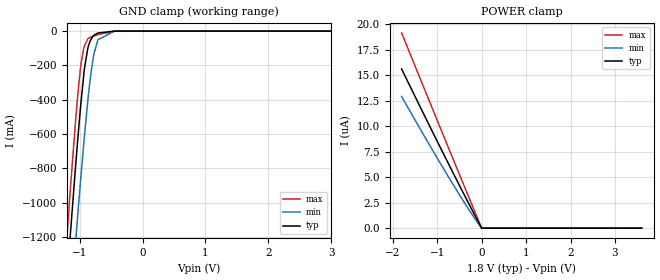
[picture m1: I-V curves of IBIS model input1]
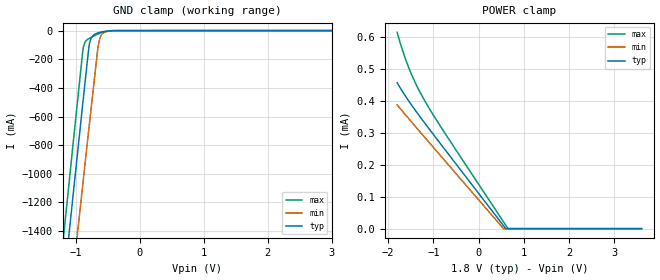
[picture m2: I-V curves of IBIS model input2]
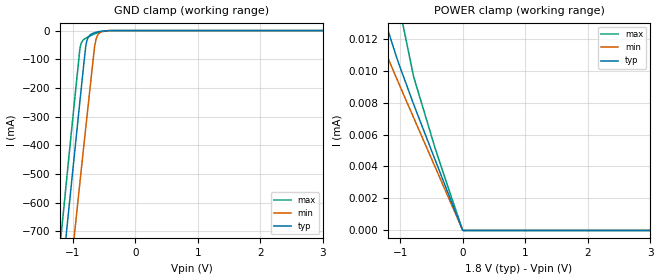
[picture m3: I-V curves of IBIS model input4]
| Texas Instruments Incorporated
| ADS92xx
| 2-Channel, 16/18-Bit, 5/10-MSPS SAR ADC
| With Integrated Driver for the ADC inputs
[IBIS Ver]   4.1
[File name]   ads92xx.ibs
[File Rev]   1.0
[Date]   26/12/2023
[Source]
| Texas Instruments Incorporated.
| Analog-eLab Design Center, HPA
| 12500 TI Blvd
| Dallas, TX -75243
[Notes]   Revision History:
| Rev 1.0: 26/12/2023
| - Initial version of the model
| - Model generated from simulations in SPECTRE
| - Model matched to SPICE simulation
| - C_comp although listed in numerical order of value are
|   obtained from varying PVT conditions. For PVT conditions for
|   each specific value refer the buffer description under
|   respective [Model]. IBIS model user is responsible for using
|   appropriate C_comp to simulate for Signal Integrity.
| - Warnings regarding combined Non-monotonicity of various models have been
|   reviewed and considered minor and can be ignored.
[Disclaimer]
| This model is designed as an aid for customers of Texas Instruments.
| TI and its licensors and suppliers make no warranties, either expressed
| or implied, with respect to this  model, including the warranties of
| merchantability or fitness for a particular purpose. The model is
| provided solely on an "as is" basis. The entire risk as to its quality
| and performance is with the customer.
[Copyright]
(C) Copyright 2023 Texas Instruments Incorporated.All rights reserved.
|   ADS9227, ADS9228, ADS9218
[Component]   ADS92xx
[Manufacturer]   TI
[Package]   |40 VQFN
|   typ   min   max
R_pkg   0.08   0.04   0.12
L_pkg   1.2nH   0.6nH   1.8nH
C_pkg   0.17pF   0.14pF   0.20pF
[Pin] signal_name  model_name   R_pin   L_pin   C_pin
1   AVDD_5V   power   NA   NA   NA
2   GND   gnd   NA   NA   NA
3   AINAP   nc   NA   NA   NA
4   AINAM   nc   NA   NA   NA
5   VCMOUT   nc   NA   NA   NA
6   REFM   nc   NA   NA   NA
7   AINBP   nc   NA   NA   NA
8   AINBM   nc   NA   NA   NA
9   GND   gnd   NA   NA   NA
10   AVDD_5V   power   NA   NA   NA
11   REFM   nc   NA   NA   NA
12   GND   gnd   NA   NA   NA
13   VDD_1V8   power   NA   NA   NA
14   VDD_1V8   power   NA   NA   NA
15   GND   gnd   NA   NA   NA
16   SPI_EN   input1   NA   NA   NA
17   CSz   input1   NA   NA   NA
18   SCLK   input4   NA   NA   NA
19   SDI   input4   NA   NA   NA
20   SDO   output1   NA   NA   NA
21   RESETz   input4   NA   NA   NA
22   PWDNz   input4   NA   NA   NA
23   DCLKM   diffout   NA   NA   NA
24   DCLKP   diffout   NA   NA   NA
25   DOUTBM   diffout   NA   NA   NA
26   DOUTBP   diffout   NA   NA   NA
27   DOUTAM   diffout   NA   NA   NA
28   DOUTAP   diffout   NA   NA   NA
29   FCLKM   diffout   NA   NA   NA
30   FCLKP   diffout   NA   NA   NA
31   SMPL_CLKM   input2   NA   NA   NA
32   SMPL_CLKP   input2   NA   NA   NA
33   SMPL_SYNC   input5   NA   NA   NA
34   GND   gnd   NA   NA   NA
35   VDD_1V8   power   NA   NA   NA
36   VDD_1V8   power   NA   NA   NA
37   VDD_1V8   power   NA   NA   NA
38   GND   gnd   NA   NA   NA
39   REFIO   nc   NA   NA   NA
40   REFM   nc   NA   NA   NA
[Diff pin]  inv_pin  vdiff  tdelay_typ  tdelay_min  tdelay_max
24   23   0.0   0.0s   0.0s   0.0s
26   25   0.0   0.0s   0.0s   0.0s
28   27   0.0   0.0s   0.0s   0.0s
30   29   0.0   0.0s   0.0s   0.0s
| Models and submodels in the file (6): input1 (Input), input2 (Input), input4 (Input), input5 (Input), output1 (3-state), diffout (3-state)
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|   input1 Model
[Model]   input1
Model_type   Input
Vinl = 0.54
Vinh = 1.26
|   typ   min   max
C_comp   0.672pF   0.636pF   0.697pF
[Voltage Range]   1.8   1.75   1.85
[Temperature Range]   27   125   -40
[Power Clamp Reference]   1.8   1.75   1.85
[GND Clamp Reference]   0   0   0
[GND Clamp]
|   Voltage   I(typ)   I(min)   I(max)
-1.8V     -4.321A    -4.211A    -4.387A
-1.195V   -1.418A    -1.849A    -1.162A
-1.147V   -1.178A    -1.615A    -916mA
-1.044V   -693.2mA   -1.134A    -431.7mA
-984.6mV  -438.2mA   -867.3mA   -208.3mA
-936mV    -259.3mA   -660.5mA   -102.1mA
-871.2mV  -101.4mA   -409.6mA   -46.07mA
-838.8mV  -63.14mA   -300.5mA   -37.3mA
-774mV    -23.82mA   -134.1mA   -29.01mA
-709.2mV  -11.34mA   -50.08mA   -20.86mA
-444.6mV  -226.7uA   -207uA     -338.8uA
3.6V      0A         0A         0A
[POWER Clamp]
|   Voltage   I(typ)   I(min)   I(max)
-1.8V     15.62uA    12.93uA    19.16uA
-1.222V   10.49uA    8.533uA    12.96uA
-720mV    6.094uA    4.84uA     7.608uA
-309.6mV  2.579uA    1.973uA    3.258uA
-1.8mV    10.88nA    7.532nA    14.89nA
3.6V      0A         0A         0A
|   input2 Model
[Model]   input2
Model_type   Input
Vinl = 0.54
Vinh = 1.26
|   typ   min   max
C_comp   1.84pF   1.72pF   2.03pF
[Voltage Range]   1.8   1.75   1.85
[Temperature Range]   27   125   -40
[Power Clamp Reference]   1.8   1.75   1.85
[GND Clamp Reference]   0   0   0
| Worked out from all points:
|   GND clamp passes 1 mA (typ) near -0.44 V on its own axis
[GND Clamp]
|   Voltage   I(typ)   I(min)   I(max)
-1.8V     -4.415A    -4.911A    -4.109A
-1.33V    -2.396A    -2.926A    -2.058A
-1.12V    -1.494A    -2.04A     -1.141A
-1.055V   -1.218A    -1.769A    -859.4mA
-1.006V   -1.011A    -1.566A    -648.9mA
-882mV    -486.1mA   -1.051A    -125.9mA
-784.8mV  -96.7mA    -656.1mA   -54.09mA
-709.2mV  -27.49mA   -351.2mA   -36.6mA
-649.8mV  -16.05mA   -116.8mA   -24.29mA
-622.8mV  -12.53mA   -57.25mA   -19.32mA
-536.4mV  -4.706mA   -7.688mA   -7.279mA
3.6V      0A         0A         0A
[POWER Clamp]
|   Voltage   I(typ)   I(min)   I(max)
-1.8V     456.5uA    387.1uA    614uA
-1.681V   428.7uA    366.9uA    557.6uA
-1.611V   413.4uA    355.2uA    528.6uA
-1.508V   392.1uA    338.1uA    491.1uA
-1.336V   358uA      309.5uA    438uA
-1.179V   328.2uA    283.7uA    397.1uA
-790.2mV  255.9uA    219.8uA    308.4uA
549mV     9.364uA    174.3nA    21.56uA
597.6mV   426.3nA    0A         11.18uA
646.2mV   0A         0A         795.4nA
3.6V      0A         0A         0A
|   input4 Model
[Model]   input4
Model_type   Input
Vinl = 0.54
Vinh = 1.26
|   typ   min   max
C_comp   0.383pF   0.369pF   0.397pF
[Voltage Range]   1.8   1.75   1.85
[Temperature Range]   27   125   -40
[Power Clamp Reference]   1.8   1.75   1.85
[GND Clamp Reference]   0   0   0
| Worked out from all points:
|   GND clamp passes 1 mA (typ) near -0.48 V on its own axis
[GND Clamp]
|   Voltage   I(typ)   I(min)   I(max)
-1.8V     -2.211A    -2.457A    -2.059A
-1.082V   -666.2mA   -940.9mA   -487.6mA
-1.001V   -493.3mA   -771.4mA   -311.3mA
-882mV    -241.6mA   -524.9mA   -61.23mA
-855mV    -185.2mA   -469.4mA   -40.08mA
-784.8mV  -47.19mA   -326.8mA   -25.75mA
-757.8mV  -25.6mA    -272.2mA   -22.63mA
-709.2mV  -12.91mA   -174.2mA   -17.31mA
-649.8mV  -7.402mA   -57.4mA    -11.39mA
-622.8mV  -5.724mA   -27.78mA   -9.01mA
-536.4mV  -2.04mA    -3.437mA   -3.272mA
3.6V      0A         0A         0A
[POWER Clamp]
|   Voltage   I(typ)   I(min)   I(max)
-1.8V     29.43uA    17.45uA    104.2uA
-1.379V   15.38uA    12.52uA    31.27uA
-1.26V    13.44uA    11.38uA    23.11uA
-1.179V   12.32uA    10.63uA    19.25uA
-1.012V   10.31uA    9.097uA    13.93uA
-784.8mV  7.891uA    7.052uA    9.614uA
-444.6mV  4.447uA    3.999uA    5.187uA
-1.8mV    16nA       28.77nA    19.1nA
3.6V      0A         0A         0A
